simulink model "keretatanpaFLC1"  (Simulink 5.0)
settings: Solver=ode45  StartTime=0.0  StopTime=300  RelTol=1e-6

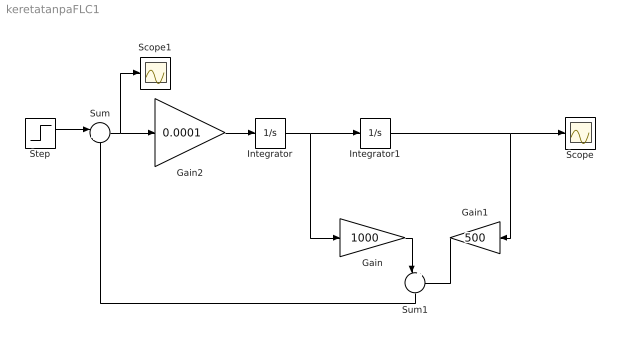
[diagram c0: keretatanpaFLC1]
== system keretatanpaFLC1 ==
  Gain : Gain  Gain=1000
  Gain1 : Gain  Orientation=left  Gain=500
  Gain2 : Gain  Gain=0.0001
  Integrator : Integrator
  Integrator1 : Integrator
  Scope : Scope
  Scope1 : Scope
  Step : Step  Time=0  After=500  SampleTime=0
  Sum : Sum  Inputs=|+-
  Sum1 : Sum  Orientation=down  Inputs=|++
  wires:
  Integrator1/1 -> Gain1/1, Scope/1
  Integrator/1 -> Integrator1/1, Gain/1
  Gain2/1 -> Integrator/1
  Sum/1 -> Gain2/1, Scope1/1
  Step/1 -> Sum/1
  Gain1/1 -> Sum1/2
  Gain/1 -> Sum1/1
  Sum1/1 -> Sum/2
